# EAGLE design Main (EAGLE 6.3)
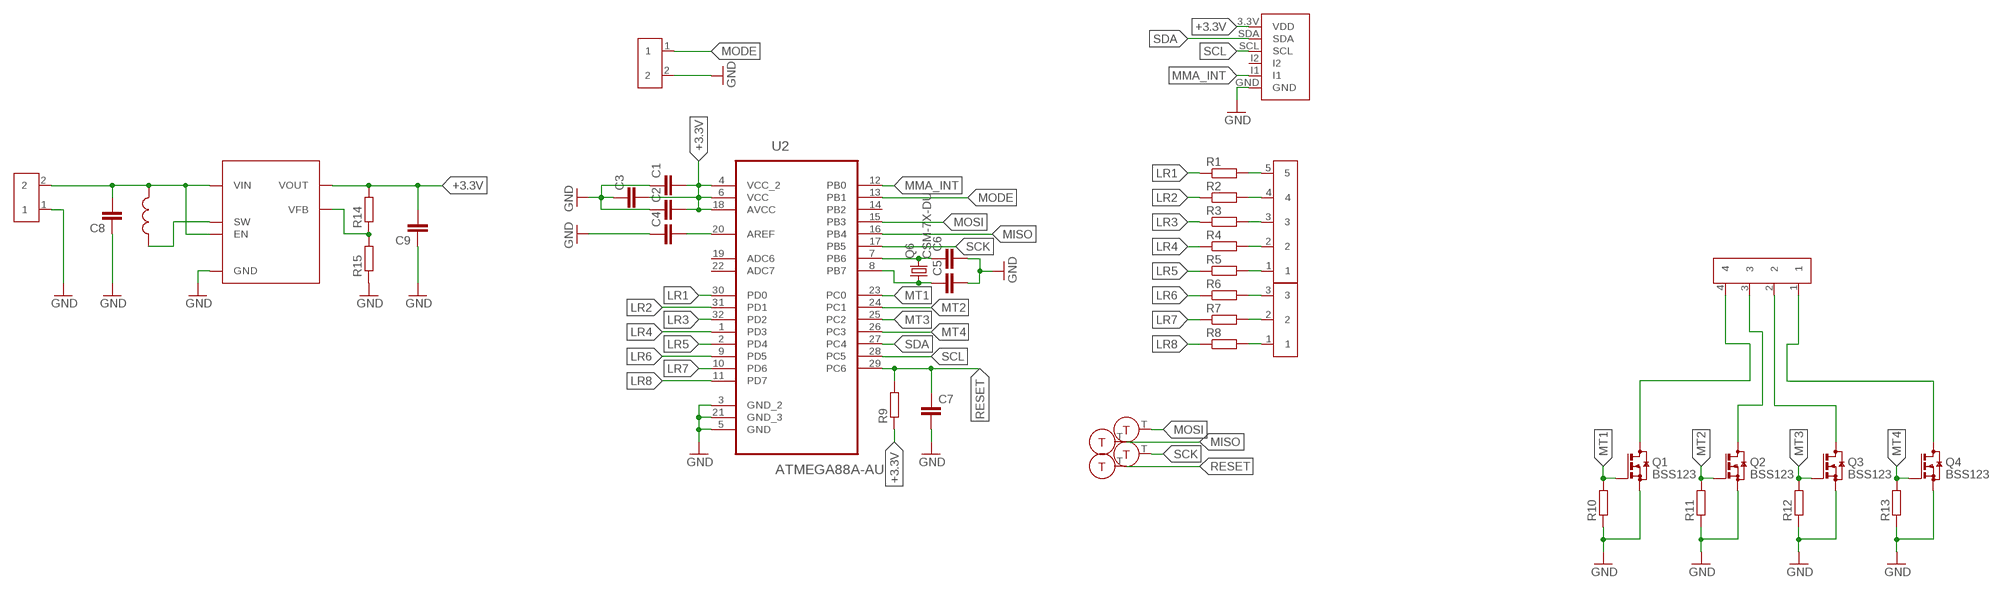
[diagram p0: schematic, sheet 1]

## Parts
C1  C-EUC0805  [C0805]
C2  C-EUC0805  [C0805]
C3  C-EUC0805  [C0805]
C4  C-EUC0805  [C0805]
C5  C-EUC0805  [C0805]
C6  C-EUC0805  [C0805]
C7  C-EUC0805  [C0805]
C8  C-EUC0805  [C0805]
C9  C-EUC0805  [C0805]
Q1  BSS123  [SOT23]
Q2  BSS123  [SOT23]
Q3  BSS123  [SOT23]
Q4  BSS123  [SOT23]
Q6  CSM-7X-DU  [CSM-7X-DU]
R1  R-EU_M0805  [M0805]
R2  R-EU_M0805  [M0805]
R3  R-EU_M0805  [M0805]
R4  R-EU_M0805  [M0805]
R5  R-EU_M0805  [M0805]
R6  R-EU_M0805  [M0805]
R7  R-EU_M0805  [M0805]
R8  R-EU_M0805  [M0805]
R9  R-EU_M0805  [M0805]
R10  R-EU_M0805  [M0805]
R11  R-EU_M0805  [M0805]
R12  R-EU_M0805  [M0805]
R13  R-EU_M0805  [M0805]
R14  R-EU_M0805  [M0805]
R15  R-EU_M0805  [M0805]
U2  ATMEGA88A-AU  [QFP80P900X900X120-32N]
U$1  MMA8452Q  [MMA8452Q]
U$2  WS-02S  [WS-02S]
U$14  MCP1640  [SOT23-6]
U$15  DLJ3015  [DLJ3015]
U$16  TEST_POINT  [TEST_POINT]
U$17  TEST_POINT  [TEST_POINT]
U$18  TEST_POINT  [TEST_POINT]
U$19  TEST_POINT  [TEST_POINT]
U$20  WS-02S  [WS-02S]
U$21  WS-03S  [WS-03S]
U$22  WS-04S  [WS-04S]
U$23  WS-05S  [WS-05S]

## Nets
+3.3V: C1.2 C2.2 C3.2 C9.2 R9.1 R14.2 U2.4(VCC_2) U2.6(VCC) U2.18(AVCC) U$1.3.3V(VDD) U$14.5(VOUT)
GND: C1.1 C2.1 C3.1 C4.1 C5.2 C6.2 C7.2 C8.1 C9.1 Q1.2(S) Q2.2(S) Q3.2(S) Q4.2(S) R10.1 R11.1 R12.1 R13.1 R15.1 U2.3(GND_2) U2.5(GND) U2.21(GND_3) U$1.GND U$2.1 U$14.2(GND) U$20.2
LR1: R1.1 U2.30(PD0)
LR2: R2.1 U2.31(PD1)
LR3: R3.1 U2.32(PD2)
LR4: R4.1 U2.1(PD3)
LR5: R5.1 U2.2(PD4)
LR6: R6.1 U2.9(PD5)
LR7: R7.1 U2.10(PD6)
LR8: R8.1 U2.11(PD7)
MISO: U2.16(PB4) U$17.T
MMA_INT: U2.12(PB0) U$1.I1
MODE: U2.13(PB1) U$20.1
MOSI: U2.15(PB3) U$16.T
MT1: Q1.1(G) R10.2 U2.23(PC0)
MT2: Q2.1(G) R11.2 U2.24(PC1)
MT3: Q3.1(G) R12.2 U2.25(PC2)
MT4: Q4.1(G) R13.2 U2.26(PC3)
N$1: R1.2 U$23.5
N$2: R2.2 U$23.4
N$3: C4.2 U2.20(AREF)
N$4: C6.1 Q6.2 U2.7(PB6)
N$5: C5.1 Q6.1 U2.8(PB7)
N$6: R3.2 U$23.3
N$7: R4.2 U$23.2
N$8: R5.2 U$23.1
N$9: C8.2 U$2.2 U$14.3(EN) U$14.6(VIN) U$15.P$2
N$10: R6.2 U$21.3
N$11: R7.2 U$21.2
N$12: R8.2 U$21.1
N$13: Q1.3(D) U$22.4
N$14: Q2.3(D) U$22.3
N$15: Q3.3(D) U$22.2
N$16: Q4.3(D) U$22.1
N$17: U$14.1(SW) U$15.P$1
N$18: R14.1 R15.2 U$14.4(VFB)
RESET: C7.1 R9.2 U2.29(PC6) U$19.T
SCK: U2.17(PB5) U$18.T
SCL: U2.28(PC5) U$1.SCL
SDA: U2.27(PC4) U$1.SDA
Unconnected: U2.14(PB2) U2.19(ADC6) U2.22(ADC7) U$1.I2

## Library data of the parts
C1-C9 = rcl:C-EU: CAPACITOR, European symbol
Q1-Q4 = transistor-small-signal:BSS123: N-CHANNEL MOS FET
Q6 = crystal:CSM-7X-DU: SMD CRYSTAL; OC_FARNELL: unknown; OC_NEWARK: unknown
R1-R15 = rcl:R-EU_: RESISTOR, European symbol
U2 = Atmel_By_element14_Batch_1-00:ATMEGA88A-AU: MCU; DESCRIPTION: MCU; MPN: ATMEGA88A-AU; OC_FARNELL: 1841614; OC_NEWARK: 12T1303; PACKAGE: QFP-32; SUPPLIER: Atmel
U$1 = Mario:MMA8452Q
U$2 U$20 = Mario:WS-02S
U$14 = Mario:MCP1640
U$15 = Mario:DLJ3015
U$16-U$19 = Mario:TEST_POINT
U$21 = Mario:WS-03S
U$22 = Mario:WS-04S
U$23 = Mario:WS-05S

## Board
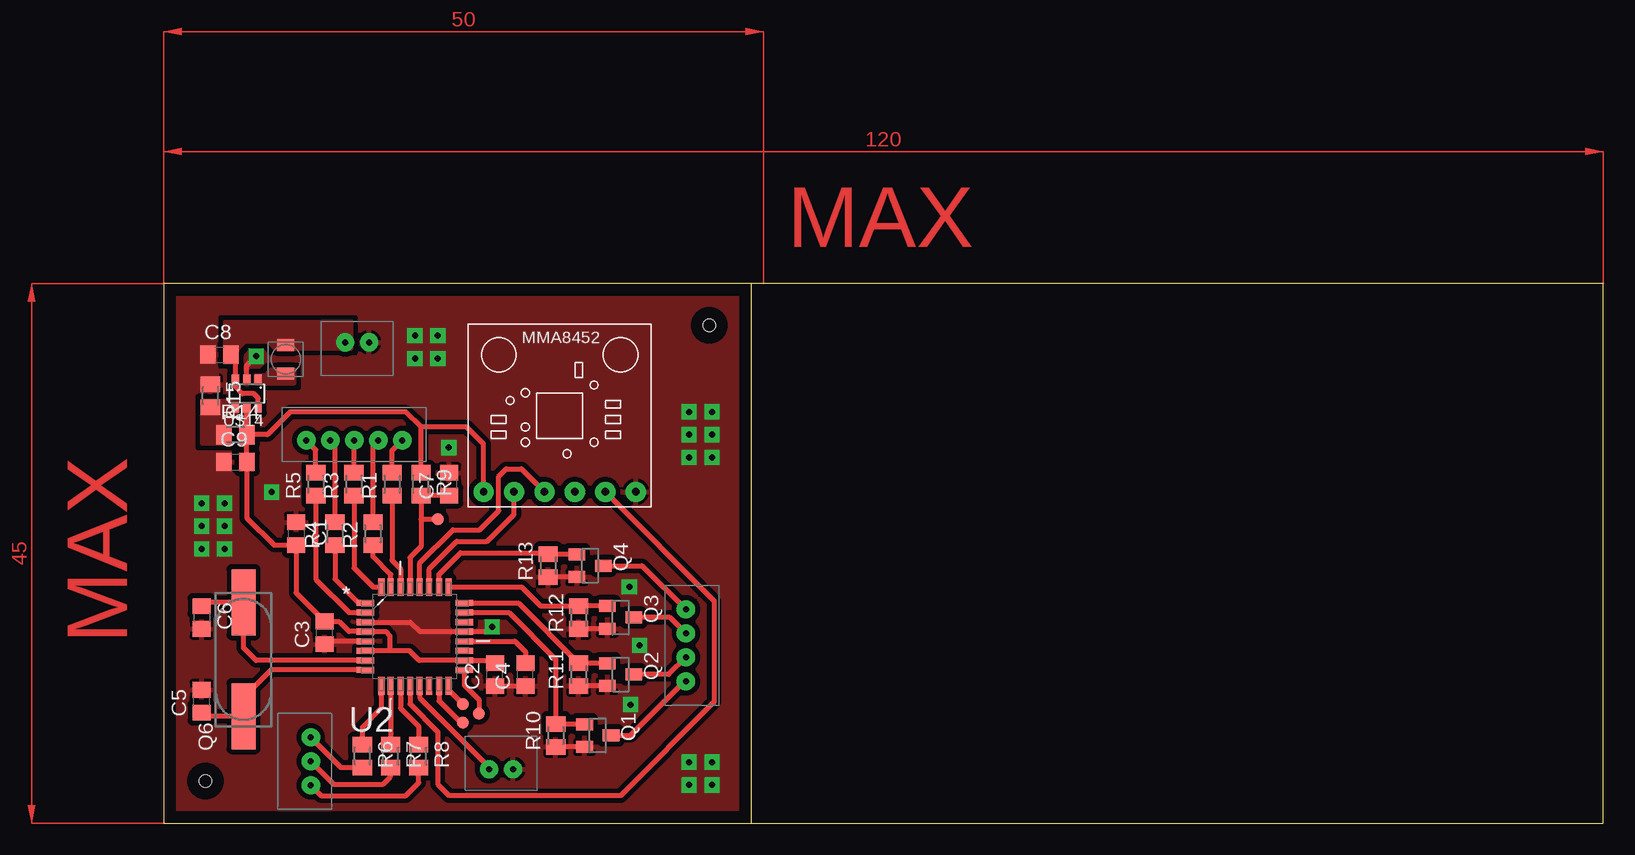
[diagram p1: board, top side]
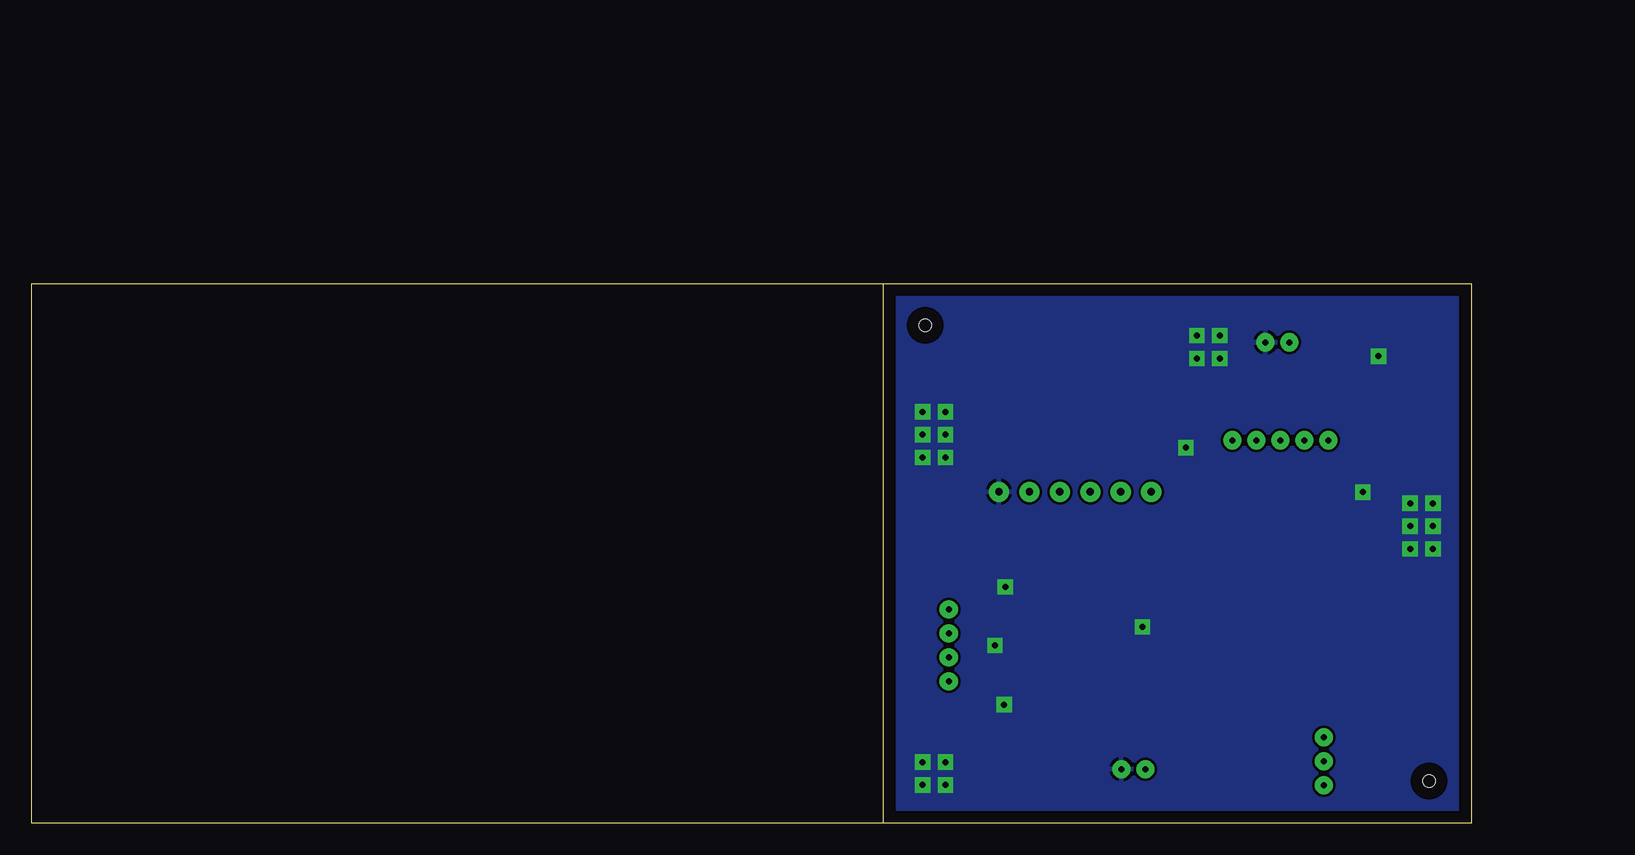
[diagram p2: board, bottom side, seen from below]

Size 120 x 45 mm. Coordinates in mm from the lower left corner, seen from the top.
Outline: 49,0 0,0 0,45 49,45
Outline: 49,0 120,0 120,45 49,45
Outline: 49,0 49,45
Copper layers (1*16): Top 0.035mm / dielectric 1.5mm / Bottom 0.035mm
Design rules "default": minimum track width 10mil, minimum drill 24mil, track to track 8mil, track to pad 8mil, pad to pad 8mil, via to via 8mil, smd to smd 8mil, copper to edge 40mil, drill to drill 8mil, minimum pad ring 10mil, minimum via ring 8mil, stop-mask expansion 4mil, vias tented up to drill 0mil, thermal gap 10mil
Holes 1 mm at 3.5,3.5 45.5,41.5

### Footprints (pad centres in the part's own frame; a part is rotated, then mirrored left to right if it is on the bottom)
C0805 = smd 1.3 x 1.5: 1 -0.95,0; 2 0.95,0
SOT23 = smd 1 x 1.4: 1 -0.95,-1.1; 2 0.95,-1.1; 3 0,1.1
CSM-7X-DU = smd 5.5 x 2: 1 -4.75,0; 2 4.75,0
M0805 = smd 1.3 x 1.6: 1 -0.95,0; 2 0.95,0
QFP80P900X900X120-32N = smd 1.473 x 0.508: 1 -4.115,2.794; 2 -4.115,2.007; 3 -4.115,1.194; 4 -4.115,0.406; 5 -4.115,-0.406; 6 -4.115,-1.194; 7 -4.115,-2.007; 8 -4.115,-2.794; 17 4.115,-2.794; 18 4.115,-2.007; 19 4.115,-1.194; 20 4.115,-0.406; 21 4.115,0.406; 22 4.115,1.194; 23 4.115,2.007; 24 4.115,2.794 | smd 0.508 x 1.473: 9 -2.794,-4.115; 10 -2.007,-4.115; 11 -1.194,-4.115; 12 -0.406,-4.115; 13 0.406,-4.115; 14 1.194,-4.115; 15 2.007,-4.115; 16 2.794,-4.115; 25 2.794,4.115; 26 2.007,4.115; 27 1.194,4.115; 28 0.406,4.115; 29 -0.406,4.115; 30 -1.194,4.115; 31 -2.007,4.115; 32 -2.794,4.115
MMA8452Q = drill 0.6 pad 1.676: 3.3V -6.35,-6.35; GND 6.35,-6.35; I1 3.81,-6.35; I2 1.27,-6.35; SCL -1.27,-6.35; SDA -3.81,-6.35
WS-02S = drill 0.5 pad 1.524: 1 2,-2.75; 2 4,-2.75
SOT23-6 = smd 0.6 x 0.9: 1 -0.95,-1.15; 2 0,-1.15; 3 0.95,-1.15; 4 0.95,1.15; 5 0,1.15; 6 -0.95,1.15
DLJ3015 = smd 1 x 1.4: P$1 -1.2,0; P$2 1.2,0
TEST_POINT = smd 1.016 x 1.016: T 0,0
WS-03S = drill 0.5 pad 1.524: 1 2,-2.75; 2 4,-2.75; 3 6,-2.75
WS-04S = drill 0.5 pad 1.524: 1 2,-2.75; 2 4,-2.75; 3 6,-2.75; 4 8,-2.75
WS-05S = drill 0.5 pad 1.524: 1 2,-2.75; 2 4,-2.75; 3 6,-2.75; 4 8,-2.75; 5 10,-2.75

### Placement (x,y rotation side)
C1  11.05,24.13 270 top
C2  27.62,12.38 90 top
C3  13.43,15.86 90 top
C4  30.16,12.38 90 top
C5  3.17,10.16 90 top
C6  3.17,17.14 270 top
C7  23.81,28.26 90 top
C8  4.67,39.05 0 top
C9  6,30.1 0 top
Q1  36.2,7.3 270 top
Q2  38.1,12.38 270 top
Q3  38.1,17.14 270 top
Q4  35.56,21.46 270 top
Q6  6.67,13.65 90 top
R1  19.05,28.26 90 top
R2  17.46,24.13 90 top
R3  15.88,28.26 90 top
R4  14.29,24.13 90 top
R5  12.7,28.26 90 top
R6  16.57,5.59 270 top
R7  18.92,5.59 270 top
R8  21.27,5.59 270 top
R9  21.46,28.26 270 top
R10  32.7,7.3 90 top
R11  34.61,12.38 90 top
R12  34.61,17.14 90 top
R13  32.07,21.46 90 top
R14  6,32.38 0 top
R15  3.91,35.62 270 top
U2  20.95,15.56 0 top
U$1  33.02,33.97 0 top
U$2  19.15,37.34 180 top
U$14  6.95,35.81 180 top
U$15  10.19,38.67 90 top
U$16  24.96,8.38 0 top
U$17  24.96,9.91 0 top
U$18  26.29,9.14 0 top
U$19  22.86,25.34 0 top
U$20  25.15,7.24 0 top
U$21  9.53,1.14 90 top
U$22  46.29,19.81 270 top
U$23  9.91,34.67 0 top

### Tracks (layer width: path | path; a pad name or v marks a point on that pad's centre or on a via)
+3.3V
  Top 0.406: C2.2 27.4,13.55 U2.18 21.31,13.55 20.5,14.36 18.86,14.36 | R14.2 C9.2 6.95,25.43 9.21,23.18 C1.2 11.05,19.2 C3.2 13.48,16.76 14.67,16.76 15.47,15.96 U2.4 18.52,15.96 18.86,15.62 18.86,14.36 | 18.86,14.36 U2.6 | U$1.3.3V 26.67,31.62 25.27,33.02 21.46,33.02 | R14.2 U$14.5 | R9.1 21.46,33.02 | 21.46,33.02 20.19,34.29 10.57,34.29 8.67,32.38 R14.2
GND  (via drill 0.5 pad 1.27)
  Top 0.406: Q3.2 R12.1 | Q2.2 R11.1 | Q1.2 R10.1 | U$14.2 6.95,38.16 v7.71,38.92 | C2.1 C4.1 | Q4.2 R13.1 | v27.4,16.35 27.01,15.96 U2.21 21.37,15.96 20.59,16.75 U2.3 | U2.5 13.67,15.15 C3.1
  other vias: 38.83,19.68 39.69,14.83 38.93,9.87 23.78,31.31 9.02,27.59 3.17,26.67 5.08,26.67 5.08,24.77 5.08,22.86 3.17,22.86 3.17,24.77 45.72,34.29 43.81,34.29 43.81,32.38 43.81,30.48 45.72,30.48 45.72,32.38 20.95,40.64 20.95,38.73 22.86,38.73 22.86,40.64 45.72,3.17 43.81,3.17 45.72,5.08 43.81,5.08
  pour Bottom (rank 2): -3,48 123,48 123,-3 -3,-3
  pour Top (isolate 0.406, rank 2): -1,46 121,46 121,-1 -1,-1
  pour Top (isolate 0.406, no thermals): 4.57,37.15 4.38,38.39 4.38,41.05 2.19,41.05 2.19,36 4.57,36
  pour Top (isolate 0.406, no thermals): 5.62,30.96 3.14,30.96 3.14,28.29 6,28.29 6,28.96 5.62,29.34
LR1
  Top 0.406: R1.1 19.05,21.91 19.76,21.2 U2.30
LR2
  Top 0.406: U2.31 18.95,20.74 17.46,22.23 R2.1
LR3
  Top 0.406: R3.1 15.88,21.27 17.48,19.67 U2.32
LR4
  Top 0.406: R4.1 14.29,20.32 16.19,18.41 16.78,18.41 U2.1
LR5
  Top 0.406: R5.1 12.7,20.32 15.46,17.56 U2.2
LR6
  Top 0.406: U2.9 18.16,9.59 16.57,8 R6.1
LR7
  Top 0.406: U2.10 18.95,6.56 R7.1
LR8
  Top 0.406: U2.11 19.76,9.58 21.27,8.06 R8.1
MISO
  Top 0.406: U2.16 23.75,11.11 U$17.T
MMA_INT
  Top 0.406: U2.12 20.55,9.93 22.86,7.62 22.86,3.24 23.81,2.29 38.1,2.29 45.91,10.1 45.91,18.54 U$1.I1
MODE
  Top 0.406: U2.13 21.36,10.45 27.15,4.67 U$20.1
MOSI
  Top 0.406: U2.15 22.96,10.19 24.77,8.38 U$16.T
MT1
  Top 0.406: Q1.1 R10.2 32.7,13.65 28.79,17.56 U2.23
MT2
  Top 0.406: U2.24 29.59,18.35 R11.2 Q2.1
MT3
  Top 0.406: Q3.1 R12.2 31.43,18.09 29.86,19.67 U2.25
MT4
  Top 0.406: U2.26 22.96,20.74 24.77,22.54 31.94,22.54 R13.2 Q4.1
N$1
  Top 0.406: R1.2 19.05,31.07 U$23.5
N$2
  Top 0.406: R2.2 17.46,31.48 U$23.4
N$3
  Top 0.406: U2.20 29.3,15.15 30.16,14.29 C4.2
N$4
  Top 0.406: U2.7 7.72,13.55 6.67,14.61 Q6.2 3.48,18.4 C6.1
N$5
  Top 0.406: U2.8 8.95,12.76 6.67,10.48 Q6.1 3.48,8.9 C5.1
N$6
  Top 0.406: R3.2 15.88,31.89 U$23.3
N$7
  Top 0.406: R4.2 14.29,31.54 U$23.2
N$8
  Top 0.406: R5.2 12.7,31.13 U$23.1
N$9
  Top 0.406: C8.2 6,38.67 U$14.3 6,36.39 6.57,35.81 7.53,35.81 7.9,35.44 U$14.6
  pour Top (no thermals): 11.14,39.53 15.72,39.53 15.72,41.81 5.05,41.81 5.05,38.39 6.19,38.39 6.19,39.34 6.19,39.43 6.86,40.1 8.67,40.1 9.24,39.53
N$10
  Top 0.406: R6.2 14.78,4.64 U$21.3
N$11
  Top 0.406: R7.2 18.92,3.87 18.29,3.24 14.18,3.24 U$21.2
N$12
  Top 0.406: U$21.1 13.13,2.29 20.19,2.29 21.27,3.37 R8.2
N$13
  Top 0.406: Q1.3 38.92,7.3 43.44,11.81 U$22.4
N$14
  Top 0.406: U$22.3 42.11,12.38 Q2.3
N$15
  Top 0.406: 39.37,17.14 Q3.3 42.21,17.14 U$22.2
N$16
  Top 0.406: Q4.3 39.89,21.46 U$22.1
N$17
  pour Top (no thermals): 7.72,37.34 8.57,37.34 9.05,37.81 10.86,37.81 10.86,36.67 7.72,36.67
N$18
  pour Top (isolate 0.406, no thermals): 5.62,31.62 5.62,33.53 6.19,34.1 6.19,35.24 3.14,35.24 3.14,31.62
RESET
  Top 0.406: 21.46,25.34 R9.2 C7.1 | 21.46,25.34 21.46,23.05 20.55,22.14 U2.29 | U$19.T 21.46,25.34
SCK
  Top 0.406: U2.17 25.07,11.51 26.29,10.29 U$18.T
SCL
  Top 0.406: U2.28 21.36,21.68 24.13,24.45 26.35,24.45 27.94,26.04 27.94,28.89 28.57,29.53 29.84,29.53 U$1.SCL
SDA
  Top 0.406: U2.27 22.15,21.2 24.45,23.5 26.99,23.5 29.21,25.72 U$1.SDA
(copper drawn outside any net)
  shapes: Top area x3

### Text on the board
Top: MAX | MAX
